//DB984.AWL
// ***************************************************************************


DATA_BLOCK "XC_VERB_SR"
TITLE = Cross Coupling jobs

AUTHOR: 	SIEMENS
FAMILY: 	SISTARS7
NAME:		XCJOBDBSR
VERSION: 	4.02

//$NOW_HOW_PROTECT

//
// Datum		Name			Aktion
// ----------------------------------------------------------------------------
// 20.05.99 	Mahler		Neu

  STRUCT

	iType			: INT		:= 1;
   	iOffset 		: INT  	:= 200;
   	iLen 			: INT  	:= 50;


//#IF Default
   	iMax 			: INT  	:= 15; //Maximale Anzahl von Verbindungen dh. PCU 1 - 16
   	iAct 			: INT  	:= 15; //Aktuelle Anzahl Verbindungen
//#ENDIF

	boINIT		: BOOL;  		//VKE=1 dh. Vorbesetzung des DB984 je nach eigener PCU ausfuehren
	bOffID		: BYTE := b#16#1F;//In der Hardwarekonfig werden die IDs von 31 - 64 fuer IOS-Verbindungen
							//reserviert. Pro PCU werden zwei IDs benoetigt. Mehr wie 64 sind
							//pro CP431 nicht moeglich.  1FHexa=31

	bPCU			: BYTE := B#16#1;	//Eigene PCU-Nummer fuer Vergleich mit DB701
      bRes			: BYTE;		//Reserve

	bRVB			: BYTE := B#16#0;	//Hilfszelle Bearbeitung des Empfangs
	bRVBmax		: BYTE := B#16#3;	//Max. Anzahl Verbindungen die pro Zyklus bearbeitet werden sollen
	bSVB			: BYTE := b#16#0;	//Hilfszelle Bearbeitung des Senden
	bSVBmax		: BYTE := b#16#3;	//Max. Anzahl Verbindungen die pro Zyklus bearbeitet werden sollen

      bSec			: BYTE;		//100 ms Zaehler von 1 ... 10 dh. sec
	bMin			: BYTE;		//sec Zaehler von 1 ... 60 dh. min

      iPrtErsa		: INT;

	iKettPos		: INT  :=1;		//Postive Quittung dh. Teilanlage gestartet
	iKettNeg		: INT	 :=256;	//Negative Quittung dh. Teilanlage nicht gestartet

      auSys				: ARRAY [1..87] OF INT;    //Reserve

	auVerb			: ARRAY [1..15] OF "XC_INIT_SR_UDT";





END_STRUCT ;

BEGIN

END_DATA_BLOCK

